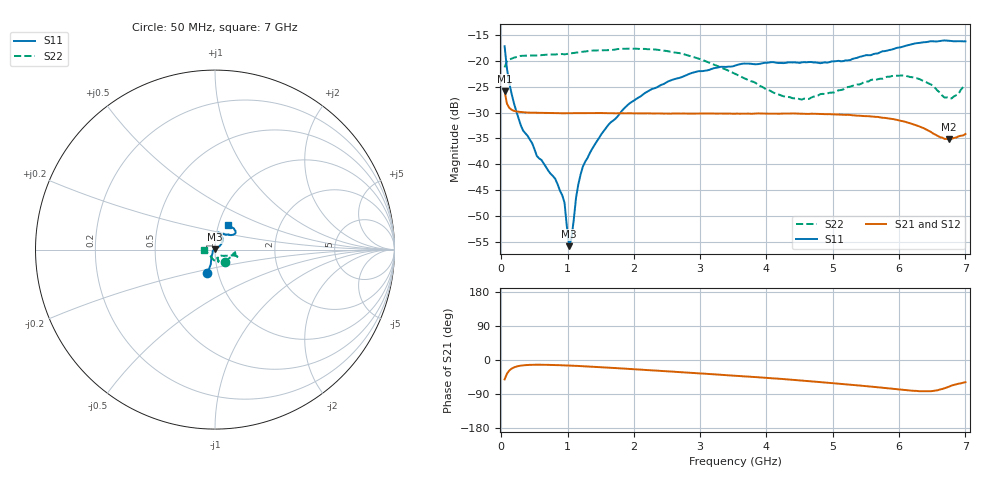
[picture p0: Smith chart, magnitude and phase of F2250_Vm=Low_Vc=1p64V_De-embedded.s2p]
! Integrated Device Technology
! Corporate Headquarters
! 6024 Silver Creek Valley Road
! San Jose, CA 95138  USA
! Phone:  1-408-284-8200
! Toll Free:  1-800-223-1366
! Webpage:  http://www.idt.com/
! Timing and RF Division
! 515 Groton Road, Suite 102
! Westford, MA 01886-6024
! Device:  F2250
! Description: Voltage Variable RF Attenuator
! Frequency:  50.0 -  6000.00 MHz
! Package:  3x3 mm Thin QFN Plastic Package: 16 pin
! Ports:  2 RF, 3 DC
!  Pin  1  = GND
!  Pin  2  = NC
!  Pin  3  = RF1  = Port 1
!  Pin  4  = NC
!  Pin  5  = GND
!  Pin  6  = GND
!  Pin  7  = GND
!  Pin  8  = GND
!  Pin  9  = NC
!  Pin 10  = RF2  = Port 2
!  Pin 11  = NC
!  Pin 12  = GND
!  Pin 13  = GND
!  Pin 14  = VCNTRL
!  Pin 15  = VDD
!  Pin 16  = VMODE
! Vcntrl:  1.640 Volts
! Vmode:  +0.000 Volts
! Vdd:  +3.30  Volts
! Current:  1.189 mA
! Data:  The device was measured on a the F2250 evaluation board which has
!  individual transmission lines to the RF pins.  Data was collected
!  using a calibrated network analyzer.  The evaluation board was
!  de-embedded using a TRL calibration technique.
!  The reference plane is the edge of the package pin.
! Misc:  SN 10
!  Action Tracker AT0258
! Date Measured:  2014-11-26
! Date:  2015-10-15  MJV
! Note:
!  Integrated Device Technology supplies this data as a sample of measured
!  data at the package pin for this product.  Your particular data for this
!  product may vary.
!  Data was taken at 25 degrees C.
!  Integrated Device Technology reserves the right to change this data at anytime.
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# GHz S dB R 50
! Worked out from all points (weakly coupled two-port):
!   201 points, 50 MHz to 7 GHz, reference 50 ohm
!   highest |S21| = -25.85 dB at 50 MHz (marker M1); lowest = -35.1 dB at 6.757 GHz (marker M2)
!   lowest |S11| = -55.9 dB at 1.023 GHz (marker M3), VSWR 1.00, Z = 49.9 + j0.123 ohm
!   |S11| at or under -10 dB: start of sweep to end of sweep
!   |S22| runs from -27.5 to -17.6 dB; largest |S21 - S12| = 0.00016
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0.05  -17.15 -107.6  -25.85 -51.2  -25.88 -51.3  -21.26 -50.7
0.1195  -24.22 -110.1  -29.09 -28.0  -29.09 -28.0  -19.73 -14.7
0.29325  -32.44 -124.2  -29.90 -14.9  -29.92 -14.9  -19.02 -8.9
0.5365  -38.42 -150.6  -30.05 -12.5  -30.05 -12.5  -18.94 -8.5
0.8145  -42.85 174.9  -30.11 -13.3  -30.12 -13.3  -18.75 -11.6
0.91875  -46.00 157.2  -30.14 -14.0  -30.13 -14.0  -18.66 -13.2
0.9535  -47.45 172.7  -30.13 -14.2  -30.13 -14.2  -18.74 -13.2
1.023  -55.89 129.6  -30.13 -14.6  -30.12 -14.6  -18.57 -13.3
1.05775  -54.44 91.2  -30.13 -14.9  -30.11 -14.9  -18.52 -13.5
1.12725  -46.54 46.1  -30.11 -15.4  -30.12 -15.4  -18.39 -14.4
1.162  -43.90 42.1  -30.12 -15.7  -30.13 -15.7  -18.33 -14.9
1.2315  -40.44 35.3  -30.10 -16.4  -30.11 -16.4  -18.19 -15.7
1.6485  -31.93 38.5  -30.13 -20.5  -30.13 -20.6  -17.90 -16.8
1.9265  -28.31 39.2  -30.13 -23.6  -30.12 -23.6  -17.63 -17.4
2.37825  -24.87 45.8  -30.18 -28.5  -30.18 -28.5  -17.86 -17.4
3.525  -20.91 71.8  -30.23 -41.4  -30.22 -41.5  -22.49 -27.4
4.25475  -20.43 77.4  -30.20 -50.3  -30.20 -50.3  -26.84 -50.0
4.7065  -20.29 71.9  -30.23 -56.7  -30.26 -56.7  -26.93 -67.7
5.85325  -17.88 40.0  -31.18 -75.2  -31.18 -75.2  -23.05 -74.7
6.305  -16.51 40.2  -32.69 -82.4  -32.68 -82.4  -23.51 -84.1
6.75675  -16.10 50.8  -35.12 -70.1  -35.12 -70.0  -27.21 -138.0
7  -16.20 62.9  -34.17 -58.7  -34.13 -58.8  -24.64 -179.6
